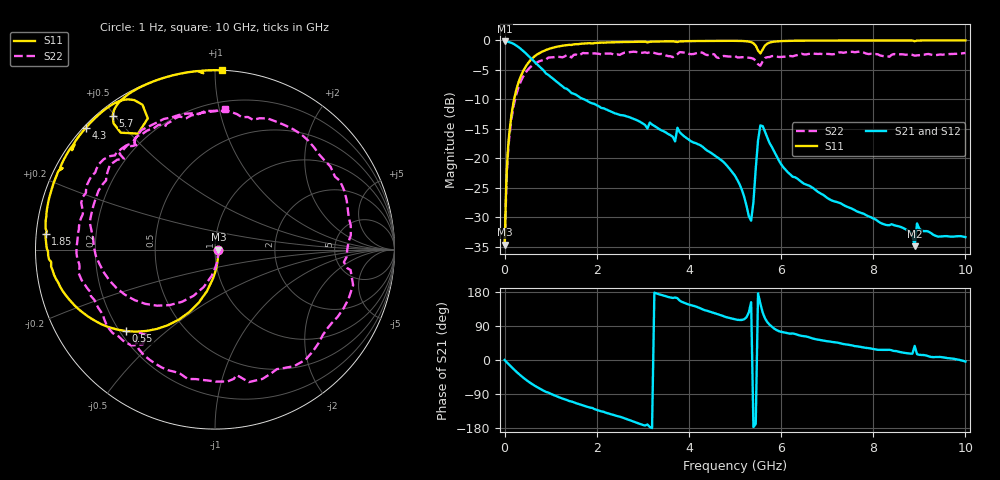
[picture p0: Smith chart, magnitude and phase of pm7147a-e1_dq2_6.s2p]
# GHz S DB R 50
! S-Parameters data
! Freq  dbS11  angS11  dbS21  angS21  dbS12  angS12  dbS22  angS22
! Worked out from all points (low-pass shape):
!   279 points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, 1 Hz to 10 GHz, reference 50 ohm
!   highest |S21| = -0.16 dB at 25.12 kHz (marker M1); lowest = -34.9 dB at 8.9 GHz (marker M2)
!   |S21| within 3 dB of the highest: start of sweep to 588.7 MHz
!   lowest |S11| = -34.7 dB at 19.95 kHz (marker M3), VSWR 1.04, Z = 51.9 - j0.00332 ohm
!   |S11| at or under -10 dB: start of sweep to 205.9 MHz
!   |S22| runs from -34.7 to -1.9 dB; largest |S21 - S12| = 0
!   S11 on the Smith chart (normalised r, x): 1 Hz: 1.04, -0.00; 550 MHz: 0.23, -0.37; 1.85 GHz: 0.03, +0.04; 4.3 GHz: 0.01, +0.40; 5.7 GHz: 0.04, +0.49; 10 GHz: 0.00, +1.04
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1e-09  -34.67 -0.0  -0.16 -0.0  -0.16 -0.0  -34.67 -0.0
1.99526e-05  -34.67 -0.1  -0.16 -0.0  -0.16 -0.0  -34.67 -0.1
2.51189e-05  -34.67 -0.1  -0.16 -0.0  -0.16 -0.0  -34.67 -0.1
0.05011872  -21.63 -82.2  -0.19 -6.3  -0.19 -6.3  -22.30 -83.2
0.15  -12.51 -101.0  -0.42 -18.6  -0.42 -18.6  -13.23 -106.8
0.55  -3.46 -137.4  -2.86 -59.8  -2.86 -59.8  -4.59 -158.7
0.95  -1.48 -158.6  -5.86 -86.0  -5.86 -86.0  -2.92 167.7
1.7  -0.53 178.4  -9.92 -119.5  -9.92 -119.5  -2.13 121.6
1.85  -0.47 174.9  -10.52 -125.6  -10.52 -125.6  -2.14 111.4
2.6  -0.27 160.9  -12.75 -153.8  -12.75 -153.8  -2.08 68.1
3.35  -0.18 149.5  -15.03 173.5  -15.03 173.5  -2.31 13.6
3.8  -0.16 143.8  -15.58 156.6  -15.58 156.6  -1.99 -14.5
4.3  -0.09 136.7  -18.06 133.5  -18.06 133.5  -2.11 -55.9
5.05  -0.07 126.5  -23.68 105.9  -23.68 105.9  -2.88 -105.7
5.35  -0.28 120.1  -30.61 152.5  -30.61 152.5  -2.99 -124.0
5.55  -2.21 123.6  -14.43 149.1  -14.43 149.1  -4.29 -128.8
5.7  -0.54 127.4  -16.46 100.0  -16.46 100.0  -2.84 -135.2
6.7  -0.03 113.1  -25.09 56.3  -25.09 56.3  -2.25 179.2
8.35  -0.01 98.9  -31.36 27.0  -31.36 27.0  -2.76 127.0
8.9  -0.13 93.8  -34.92 37.2  -34.92 37.2  -2.59 111.7
8.95  -0.03 95.2  -31.06 15.5  -31.06 15.5  -2.54 111.7
10  -0.00 87.7  -33.38 -4.1  -33.38 -4.1  -2.12 85.9
